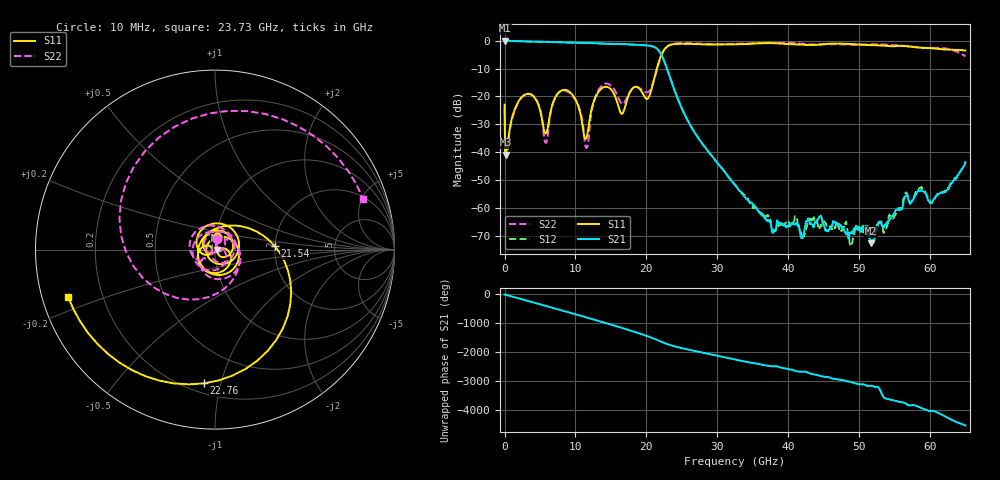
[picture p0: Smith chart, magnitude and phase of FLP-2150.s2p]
! MARKI MICROWAVE INC.
! Email:  info@markimicrowave.com  Phone:  408-778-4200
! Model Number:  FLP-2150  Date:  05/11
! Filename:		FLP-2150.S2P  Version: 1.0
! Description:  2-port S-parameter data for Low Pass Filter FLP-2150
! Features:		Low Insertion Loss, High Stop Band Rejection, Excellent Return Loss, 11th Order Filter
! Frequency Measured: 	10 MHz to 65 GHz
! Measurements:		S11, S21, S12, S22
# Hz S  dB  R 50
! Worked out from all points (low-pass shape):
!   801 points, 10 MHz to 65 GHz, reference 50 ohm
!   highest |S21| = -0.03 dB at 91.24 MHz (marker M1); lowest = -72.6 dB at 51.68 GHz (marker M2)
!   |S21| within 3 dB of the highest: start of sweep to 21.56 GHz
!   lowest |S11| = -40.8 dB at 172.5 MHz (marker M3), VSWR 1.02, Z = 50.9 - j0.165 ohm
!   |S11| at or under -10 dB: start of sweep to 21.49 GHz
!   |S22| runs from -40.0 to -0.7 dB; largest |S21 - S12| = 0.017
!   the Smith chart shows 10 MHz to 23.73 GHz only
!   S11 on the Smith chart (normalised r, x): 10 MHz: 1.01, +0.14; 21.54 GHz: 1.99, +0.09; 22.76 GHz: 0.26, -0.89; 23.73 GHz: 0.08, -0.16
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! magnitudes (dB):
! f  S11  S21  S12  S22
! 10 MHz  -22.9  0.0  0.1  -24.4
! 91.24 MHz  -40.0  0.0  0.0  -39.5
! 172.5 MHz  -40.8  0.0  0.0  -40.0
! 3.178 GHz  -19.1  -0.3  -0.3  -19.1
! 5.778 GHz  -33.3  -0.4  -0.4  -36.6
! 7.89 GHz  -18.1  -0.6  -0.6  -18.2
! 10.9 GHz  -28.7  -0.8  -0.7  -27.5
! 11.63 GHz  -34.3  -0.8  -0.8  -38.3
! 13.66 GHz  -17.2  -1.1  -1.0  -16.3
! 16.58 GHz  -26.2  -1.2  -1.2  -22.7
! 18.29 GHz  -16.7  -1.5  -1.5  -16.8
! 20.24 GHz  -20.7  -1.8  -1.8  -18.4
! 21.54 GHz  -9.6  -3.0  -3.0  -10.0
! 21.7 GHz  -8.1  -3.4  -3.4  -8.6
! 22.76 GHz  -2.5  -8.9  -8.9  -2.6
! 23.73 GHz  -1.3  -16.1  -16.1  -1.2
! 32.51 GHz  -1.3  -51.8  -51.6  -1.1
! 37.95 GHz  -0.9  -68.4  -67.6  -0.8
! 43.39 GHz  -1.6  -65.8  -63.5  -1.4
! 51.68 GHz  -1.6  -72.6  -67.1  -1.3
! 54.2 GHz  -1.9  -64.5  -62.9  -1.5
! 65 GHz  -3.6  -43.7  -43.2  -5.6
